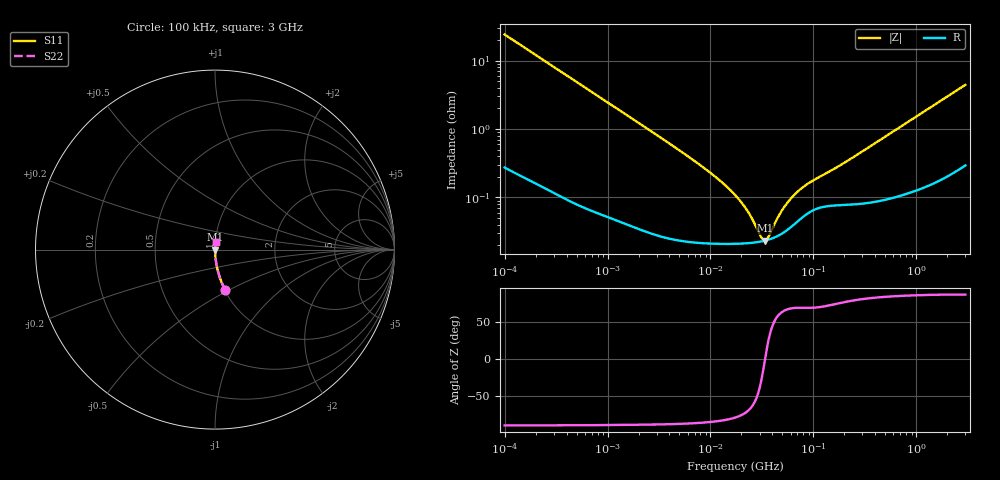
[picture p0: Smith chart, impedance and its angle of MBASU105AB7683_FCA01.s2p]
! MBASU105AB7683_FCA01  S-PARAMETER MODEL  ( Standard Model )
! Model Generated by TAIYO YUDEN Corporation (http://www.ty-top.com)
! Version 1.0
! TAIYO YUDEN Control No. 221216
! Copyright(c) 2022 TAIYO YUDEN CO.,LTD. All Rights Reserved.
! Product Description (link to TY-COMPAS)
! https://ds.yuden.co.jp/TYCOMPAS/or/detail?pn=MBASU105AB7683KFCA01&u=M
! Products Name : Multilayer Ceramic Capacitors
! Characteristics :
!  Capacitance : 0.068 [uF] , Rated Voltage : 50 [V] , TCC : X7R
!  Case Size : 1.0 x 0.5 / 0.039 x 0.02 [mm/inch] , Thickness : 0.5 / 0.02 [mm/inch]
!  (Conditions: Temperature = 25 [degC] , DC Bias Voltage = 0 [V])
! External Node Assignments :
!  1  o---| |---o  2
! GND o---------o GND
! Frequency Range : 100kHz  -  3GHz  [ 401 STEP ]
# MHZ S RI R 50
! Freq[MHz].  S11 Real  S11 Imag  S21 Real  S21 Imag  S12 Real  S12 Imag  S22 Real  S22 Imag
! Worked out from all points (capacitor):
!   401 points, 100 kHz to 3 GHz, reference 50 ohm
!   read as one part in series: C = 65.9 nF near 105.3 kHz
!   lowest |Z| = 23.4 mohm at 33.85 MHz (marker M1)
!   series resonance near 33.98 MHz, so ESL is about 330 pH
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0.1  0.0573 -0.2268  0.9427 0.2268  0.9427 0.2268  0.0573 -0.2268
0.222319  0.0132 -0.1075  0.9868 0.1075  0.9868 0.1075  0.0132 -0.1075
0.562235  0.00261 -0.0433  0.9974 0.0433  0.9974 0.0433  0.00261 -0.0433
3.161081  0.000334 -0.00778  0.9997 0.00778  0.9997 0.00778  0.000334 -0.00778
9.574722  0.000218 -0.0024  0.9998 0.0024  0.9998 0.0024  0.000218 -0.0024
13.7349  0.000212 -0.00152  0.9998 0.00152  0.9998 0.00152  0.000212 -0.00152
17.7727  0.000212 -0.00102  0.9998 0.00102  0.9998 0.00102  0.000212 -0.00102
20.74485  0.000213 -0.000759  0.9998 0.000759  0.9998 0.000759  0.000213 -0.000759
23.59795  0.000216 -0.000551  0.9998 0.000551  0.9998 0.000551  0.000216 -0.000551
31.3325  0.000228 -0.000121  0.9998 0.000121  0.9998 0.000121  0.000228 -0.000121
32.98988  0.000232 -4.38e-05  0.9998 4.38e-05  0.9998 4.38e-05  0.000232 -4.38e-05
33.85116  0.000234 -5.45e-06  0.9998 5.45e-06  0.9998 5.45e-06  0.000234 -5.45e-06
34.73492  0.000236 3.29e-05  0.9998 -3.29e-05  0.9998 -3.29e-05  0.000236 3.29e-05
36.57227  0.000242 0.00011  0.9998 -0.00011  0.9998 -0.00011  0.000242 0.00011
46.11977  0.000279 0.000463  0.9997 -0.000463  0.9997 -0.000463  0.000279 0.000463
51.12795  0.000306 0.000624  0.9997 -0.000624  0.9997 -0.000624  0.000306 0.000624
56.67997  0.000342 0.000789  0.9997 -0.000789  0.9997 -0.000789  0.000342 0.000789
73.34282  0.000473 0.0012  0.9995 -0.0012  0.9995 -0.0012  0.000473 0.0012
97.38194  0.000641 0.00162  0.9994 -0.00162  0.9994 -0.00162  0.000641 0.00162
195.2919  0.000784 0.00304  0.9992 -0.00304  0.9992 -0.00304  0.000784 0.00304
547.5153  0.00103 0.00841  0.999 -0.00841  0.999 -0.00841  0.00103 0.00841
3000  0.00487 0.0439  0.9951 -0.0439  0.9951 -0.0439  0.00487 0.0439
